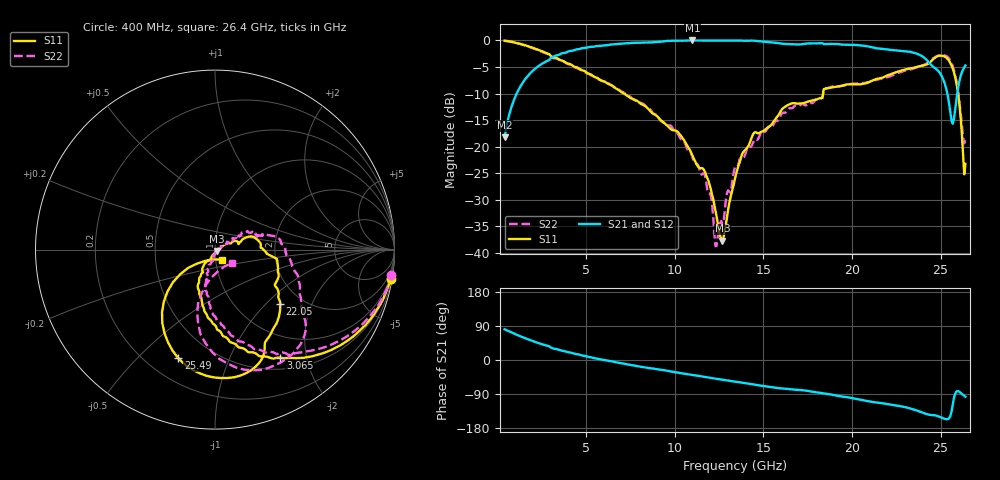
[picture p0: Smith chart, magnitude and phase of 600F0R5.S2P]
!  American Technical Ceramics  Date:  10/23/06
!  One Norden Lane
!  Huntington Station,  NY.  11746-2102
!  Tel:  (631) 622-4700  Fax:  (631) 622-4748
!  Part Number  600F0R5  Mounting Orientation: Horizontal
!  Description: Ultra Low ESR Microwave capacitors
!  Application: Coupling, Bypass, Tuning, DC Block
!  Filters, Matching
# GHZ S DB R 50
! Freq  |S11|  S11 Ph  |S21|  S21 Ph  |S12|  S12 Ph  |S22|  S22 Ph
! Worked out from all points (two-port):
!   401 points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, 400 MHz to 26.4 GHz, reference 50 ohm
!   highest |S21| = -0.01 dB at 10.99 GHz (marker M1); lowest = -18.2 dB at 400 MHz (marker M2)
!   |S21| within 3 dB of the highest: 3.195 GHz to 23.98 GHz (20.78 GHz wide, 153 % of centre)
!   lowest |S11| = -37.7 dB at 12.69 GHz (marker M3), VSWR 1.03, Z = 51 - j0.854 ohm
!   |S11| at or under -10 dB: 7.127 GHz to 18.37 GHz (11.24 GHz wide, 88.2 % of centre); 25.99 GHz to end of sweep
!   |S22| runs from -38.7 to -0.1 dB; largest |S21 - S12| = 0.0031
!   S11 on the Smith chart (normalised r, x): 400 MHz: 1, -12; 3.065 GHz: 0.66, -1.57; 22.05 GHz: 1.56, -1.21; 25.49 GHz: 0.33, -0.67; 26.4 GHz: 1.08, -0.12
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0.4  -0.07 -9.4  -18.20 81.0  -18.17 80.9  -0.06 -8.2
1.375  -0.74 -30.4  -8.20 60.9  -8.19 60.9  -0.74 -27.2
3.065  -3.06 -58.8  -3.23 31.8  -3.22 31.7  -3.08 -55.6
4.755  -5.59 -80.0  -1.47 12.0  -1.47 12.0  -5.62 -75.9
9.11  -14.64 -118.3  -0.28 -24.9  -0.29 -25.0  -14.68 -105.6
10.995  -21.66 -124.9  -0.01 -39.4  -0.01 -39.4  -21.91 -106.4
11.71  -24.78 -115.0  -0.01 -44.7  -0.01 -44.8  -25.47 -99.8
12.36  -33.09 -99.6  -0.01 -49.7  -0.01 -49.8  -38.68 -80.4
12.685  -37.68 -39.8  -0.01 -52.0  -0.01 -52.1  -34.40 19.5
13.4  -26.00 26.4  -0.01 -57.2  -0.01 -57.2  -23.90 33.9
14.505  -17.31 17.2  -0.07 -65.1  -0.09 -65.2  -18.69 29.1
17.755  -11.32 -0.5  -0.54 -83.6  -0.56 -83.6  -11.81 18.5
18.535  -9.05 -10.3  -0.69 -88.9  -0.70 -88.8  -9.02 11.1
22.045  -6.52 -39.8  -1.74 -116.5  -1.75 -116.5  -6.85 -14.1
22.11  -6.44 -40.4  -1.76 -116.9  -1.77 -116.8  -6.81 -14.5
23.865  -4.82 -58.8  -2.80 -136.7  -2.80 -136.6  -4.82 -33.0
24.58  -3.55 -67.0  -4.96 -145.3  -4.97 -145.3  -3.36 -42.1
25.1  -2.90 -87.5  -6.96 -153.1  -6.97 -153.1  -2.76 -59.9
25.49  -3.90 -108.7  -12.12 -153.3  -12.12 -153.0  -3.50 -79.8
25.685  -5.29 -121.2  -15.67 -118.0  -15.69 -118.1  -4.87 -91.6
25.945  -9.05 -138.6  -9.84 -81.9  -9.86 -82.0  -8.69 -105.7
26.4  -23.24 -54.0  -4.72 -97.0  -4.73 -97.0  -18.38 -39.4
